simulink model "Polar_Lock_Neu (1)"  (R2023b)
settings: Solver=FixedStepDiscrete  StartTime=0.0  StopTime=inf  FixedStep=0.01  RelTol=1e-3  EnableMultiTasking=on
libraries: arduinolib x6

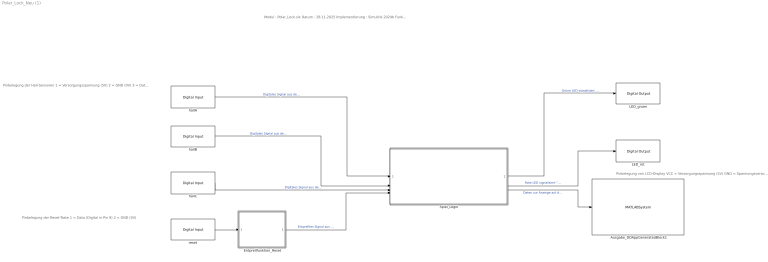
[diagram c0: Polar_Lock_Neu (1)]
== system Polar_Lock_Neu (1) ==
  note: Modul : Polar_Lock.slx Datum : 28.11.2025 Implementierung : Simulink 2024b Funktion : Steuerung von Polarlock Autor : Yash Uppal und Barinder Singh Letzte Änderung : 03.01.2026
  note: Pinbelegung von LCD-Display VCC = Versorgungsspannung (5V) GND = Spannungsversorgung, GND SDA (I/O) = Analoger Pin (A4) SCL (CLK) = Analoger Pin (A5)
  note: Pinbelegung der Hall-Sensoren 1 = Versorgungsspannung (5V) 2 = GND (0V) 3 = Data (Digitial in Pin 3, 4, 6)
  note: Pinbelegung der Reset-Taste 1 = Data (Digital in Pin 9) 2 = GND (0V)
  Ausgabe_DDAppGeneratedBlock1 : MATLABSystem  System=Ausgabe  SampleTime=-1
  Entprellfunktion_Reset : MATLAB Function  TreatAsAtomicUnit=on
  LED_gruen : arduinolib/Digital Output  pinNumber=11  Direction=output  blockPlatform=arduino
  LED_rot : arduinolib/Digital Output  pinNumber=12  Direction=output  blockPlatform=arduino
  Spiel_Logik : Subsystem
  hallA : arduinolib/Digital Input  pinNumber=3  mode=Input Pullup  Direction=input  SampleTime=0.1  blockPlatform=arduino
  hallB : arduinolib/Digital Input  pinNumber=4  mode=Input Pullup  Direction=input  SampleTime=0.1  blockPlatform=arduino
  hallC : arduinolib/Digital Input  pinNumber=6  mode=Input Pullup  Direction=input  SampleTime=0.1  blockPlatform=arduino
  reset : arduinolib/Digital Input  pinNumber=9  mode=Input Pullup  Direction=input  SampleTime=0.1  blockPlatform=arduino
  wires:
  hallA/1 -> Spiel_Logik/1(hallA)  "Digitales Signal aus dem Hall-Sensor A"
  hallB/1 -> Spiel_Logik/2(hallB)  "Digitales Signal aus dem Hall-Sensor B"
  hallC/1 -> Spiel_Logik/3(hallC)  "Digitales Signal aus dem Hall-Sensor C"
  Spiel_Logik/1(LED_gruen) -> LED_gruen/1  "Grüne LED signalisiert \"Erfolg\""
  Spiel_Logik/2(LED_rot) -> LED_rot/1  "Rote LED signalisiert \"Fehlversuch\""
  reset/1 -> Entprellfunktion_Reset/1(resetRaw)
  Entprellfunktion_Reset/1(resetDeb) -> Spiel_Logik/4(resetDeb)  "Entprelltes Signal aus der Reset-Taste"
  Spiel_Logik/3(lcdData) -> Ausgabe_DDAppGeneratedBlock1/1  "Daten zur Anzeige auf dem LCD-Display"

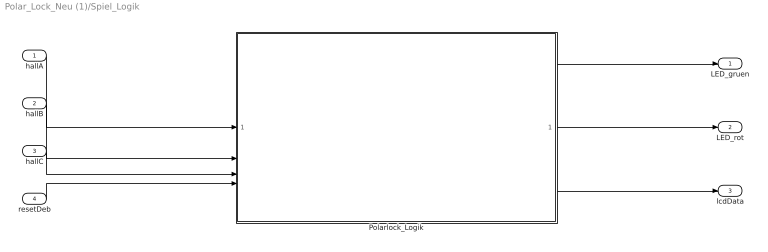
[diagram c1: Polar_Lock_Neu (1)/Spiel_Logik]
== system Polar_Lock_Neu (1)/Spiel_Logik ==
  hallA : Inport
  hallB : Inport  Port=2
  hallC : Inport  Port=3
  resetDeb : Inport  Port=4
  Polarlock_Logik : MATLAB Function  TreatAsAtomicUnit=on
  LED_gruen : Outport
  LED_rot : Outport  Port=2
  lcdData : Outport  Port=3
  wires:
  hallA/1 -> Polarlock_Logik/1(hallA)
  hallB/1 -> Polarlock_Logik/2(hallB)
  hallC/1 -> Polarlock_Logik/3(hallC)
  Polarlock_Logik/1(LED_gruen) -> LED_gruen/1
  Polarlock_Logik/2(LED_rot) -> LED_rot/1
  resetDeb/1 -> Polarlock_Logik/4(reset)
  Polarlock_Logik/3(lcdData) -> lcdData/1

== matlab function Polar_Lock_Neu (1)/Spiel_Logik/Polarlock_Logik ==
%****************************************************************
% Funktion        : Polar_Lock.slx                              *
%                                                               *
% Datum           : 28.11.2025                                  *
%                                                               *
% Betreuer        : Marc Ebmeyer                                *
%                                                               *
% Funktion        : Steuerung des Polarlocks                    *
%                                                               *
% Implementation  : Matlab R2024b                               *
%                                                               *
% Author          : Barinder Singh und Yash Uppal               *
%                                                               *
% Hardware        : Arduino Uno R3                              *
%                                                               *
% Letzte Änderung : 03.01.2026                                  *
%                                                               *
%****************************************************************

function [LED_gruen, LED_rot, lcdData] = SpielLogik(hallA, hallB, hallC, reset)

% Persistente Variablen 
persistent state;                     % Aktueller Stand des Spiels
persistent prevA prevB prevC;         % Letzte stabile Hall-Sensorwerte
persistent stableCount;               % Zähler für stabile Messungen
persistent prevReset;                 % Reset-Zustand der letzten Iteration

% Initialisierung beim ersten Funktionsaufruf
if isempty(state)
    state = int32(0);                          % STATE_IDLE
end
if isempty(prevA)
    prevA = int32(-1);
    prevB = int32(-1);
    prevC = int32(-1);
end
if isempty(stableCount)
    stableCount = int32(0);
end
if isempty(prevReset)
    prevReset = int32(0);
end

%% Zustände 
STATE_IDLE        = int32(0);        % Bereit
STATE_PRUEFE      = int32(1);        % Pruefe
STATE_ERFOLG      = int32(2);        % Erfolgreich 
STATE_FEHLVERSUCH = int32(3);        % Fehlversuch

N_STABLE = int32(50);            % 50 stabile Samples

%% Ausgänge 
LED_gruen = int32(0);
LED_rot   = int32(0);
code      = int32(0);
status    = state;

%% Initialisierung von LCD-Display 
lcdData = uint8(32 * ones(16,1));   

%% Flankenerkennung & Reset hat immer Priorität 
reset_i = int32(reset ~= 0);
resetFlanke = int32(reset_i == 1 && prevReset == 0);
prevReset = reset_i;

if resetFlanke
    state = STATE_IDLE;
    stableCount = int32(0);
    prevA = int32(-1);
    prevB = int32(-1);
    prevC = int32(-1);
end


switch state

   
    case STATE_IDLE
        LED_gruen = int32(0);
        LED_rot   = int32(0);
        code      = int32(0);
        status    = STATE_IDLE;

        % Erst starten, wenn gültige Hall-Signale anliegen
        hasSignalA = (hallA == 0) || (hallA == 1);
        hasSignalB = (hallB == 0) || (hallB == 1);
        hasSignalC = (hallC == 0) || (hallC == 1);

        if hasSignalA && hasSignalB && hasSignalC
            state = STATE_PRUEFE;
            prevA = int32(hallA);
            prevB = int32(hallB);
            prevC = int32(hallC);
            stableCount = int32(1);
        end

    %%  Überprüfung auf stabile Sensorwerte
    case STATE_PRUEFE
        status = STATE_PRUEFE;

        hasSignalA = (hallA == 0) || (hallA == 1);
        hasSignalB = (hallB == 0) || (hallB == 1);
        hasSignalC = (hallC == 0) || (hallC == 1);

        if ~(hasSignalA && hasSignalB && hasSignalC)
            stableCount = int32(0);
        else
            if (hallA == prevA) && (hallB == prevB) && (hallC == prevC)
                stableCount = stableCount + 1;
            else
                stableCount = int32(1);   
                prevA = int32(hallA);
                prevB = int32(hallB);
                prevC = int32(hallC);
            end
        end

        if stableCount >= N_STABLE
            korrektA = (hallA == 1);          % 0 = Südpol / 1 = Nordpol
            korrektB = (hallB == 1);          % 0 = Südpol / 1 = Nordpol
            korrektC = (hallC == 1);          % 0 = Südpol / 1 = Nordpol

            if korrektA && korrektB && korrektC
                state = STATE_ERFOLG;
            else
                state = STATE_FEHLVERSUCH;
            end
        end
    
    case STATE_ERFOLG                     % Die Sensorwerte entsprechen dem vorgegebenen Sollmuster = Erfolgsanzeige
        LED_gruen = int32(1);
        LED_rot   = int32(0);
        code      = int32(941);
        status    = STATE_ERFOLG;
   
    case STATE_FEHLVERSUCH              % Die Sensorwerte entsprechen nicht dem vorgegebenen Sollmuster = Fehlversuch
        LED_gruen = int32(0);
        LED_rot   = int32(1);
        code      = int32(0);
        status    = STATE_FEHLVERSUCH;
end

%% Texte auf dem LCD-Display
textStr = repmat(' ',1,16);

switch status
    case STATE_IDLE
        textStr = '    Bereit      ';
    case STATE_PRUEFE
        textStr = '   Pruefe...    ';
    case STATE_ERFOLG
        textStr = 'Erfolg! Code=941';
    case STATE_FEHLVERSUCH
        textStr = 'Fehlversuch     ';
end

for i = 1:16
    lcdData(i) = uint8(textStr(i));          % Zeichenweise Übergabe an das LCD-Display
end

end

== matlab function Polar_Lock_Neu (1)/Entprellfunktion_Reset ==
%****************************************************************
% Funktion        : Polar_Lock.slx                              *
%                                                               *
% Datum           : 28.11.2025                                  *
%                                                               *
% Betreuer        : Marc Ebmeyer                                *
%                                                               *
% Funktion        : Entprellung der Reset-Taste                 *
%                                                               *
% Implementation  : Matlab R2024b                               *
%                                                               *
% Author          : Barinder Singh und Yash Uppal               *
%                                                               *
% Hardware        : Arduino Uno R3                              *
%                                                               *
% Letzte Änderung : 03.01.2026                                  *
%                                                               *
%****************************************************************
function resetDeb = Entprellfunktion_Reset(resetRaw)



N_Entprell = int32(2);   % Entprellzeit = 20 ms

persistent cnt;            % Zähler für aufeinanderfolgende High-Samples
persistent entprellt;       %  Entprelltes Reset-Signal

if isempty(cnt)
    cnt = int32(0);
end
if isempty(entprellt)
    entprellt = int32(0);
end

%% Entprellung 
if resetRaw == 1
    if cnt < N_Entprell
        cnt = cnt + 1;
    end
else
    cnt = int32(0);
    entprellt = int32(0);
end

if cnt >= N_Entprell
    entprellt = int32(1);
end

resetDeb = entprellt;
end
